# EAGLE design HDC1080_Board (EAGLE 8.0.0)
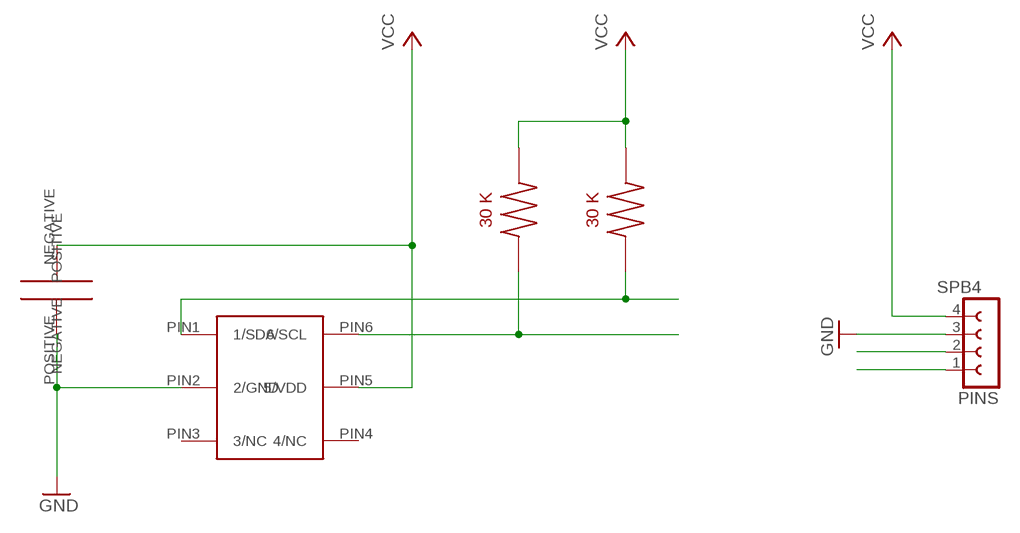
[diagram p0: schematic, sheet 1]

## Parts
PINS  SPB4  [SPB4]
U$1  HDC1080  [HDC1080]
U$2  30K_TH_RESISTOR_1135-1507  [1135-1507]
U$3  30K_TH_RESISTOR_1135-1507  [1135-1507]
U$4  CERAM_CAP_0.1UF  [CAP_CERAMIC_0.1UF]

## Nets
ONE: PINS.3 U$1.PIN2(2/GND) U$4.POSITIVE ; supply symbol labelled GND
SCL: PINS.1 U$1.PIN6(6/SCL) U$3.1
SDA: PINS.2 U$1.PIN1(1/SDA) U$2.1
VCC: PINS.4 U$1.PIN5(5/VDD) U$2.2 U$3.2 U$4.NEGATIVE
Unconnected: U$1.PIN3(3/NC) U$1.PIN4(4/NC)

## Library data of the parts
PINS = con-hirschmann:SPB4: CONNECTOR 4 pins; OC_FARNELL: unknown; OC_NEWARK: unknown
U$1 = HDC1080:HDC1080
U$2 U$3 = QBiT_Em'sComponents:30K_TH_RESISTOR_1135-1507
U$4 = Cap_Ceram_0.1uf:CERAM_CAP_0.1UF

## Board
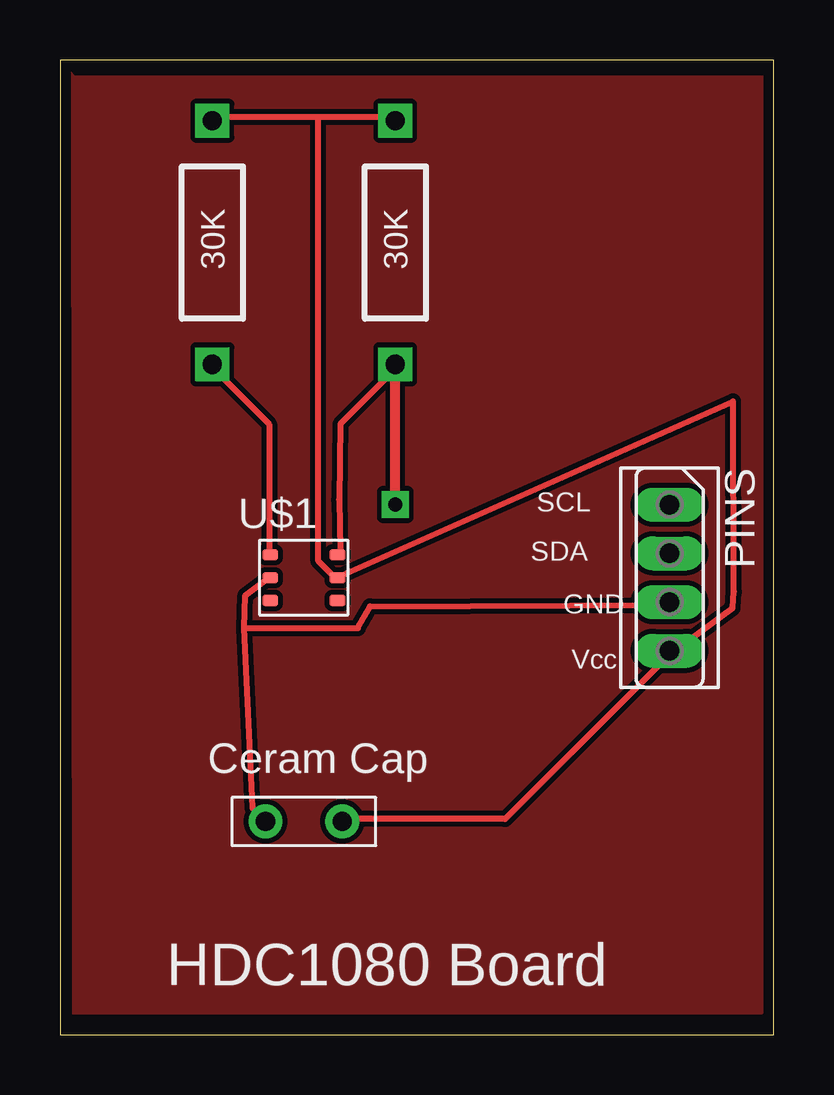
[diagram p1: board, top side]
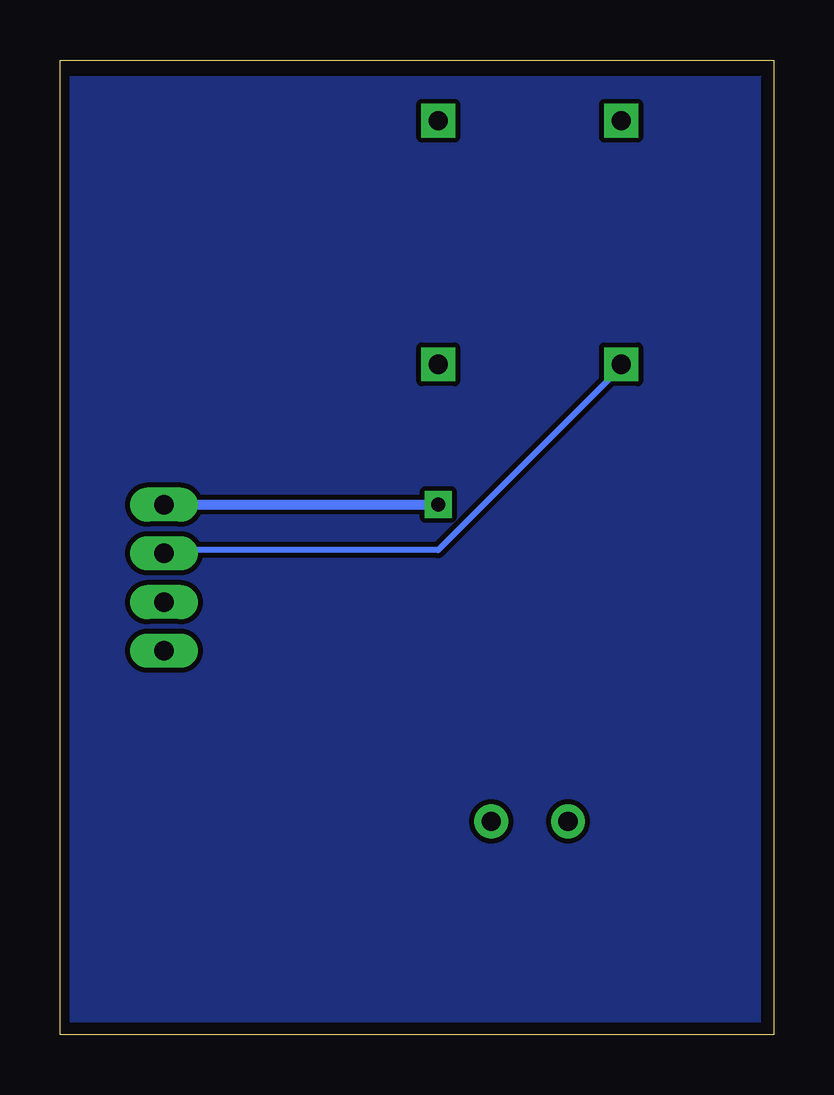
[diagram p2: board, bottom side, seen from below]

Size 29.73 x 40.63 mm. Coordinates in mm from the lower left corner, seen from the top.
Outline: 0,0 29.73,0 29.73,40.63 0,40.63 0,0
Copper layers (1*16): Top 0.035mm / dielectric 1.5mm / Bottom 0.035mm
Design rules "SparkFun": minimum track width 8mil, minimum drill 20mil, track to track 8mil, track to pad 8mil, pad to pad 8mil, via to via 8mil, smd to smd 8mil, copper to edge 10mil, drill to drill 8mil, minimum pad ring 12mil, minimum via ring 10mil, stop-mask expansion 4mil, vias tented up to drill 25mil, thermal gap 10mil

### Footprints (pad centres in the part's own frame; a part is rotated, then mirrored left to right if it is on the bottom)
SPB4 = drill 0.813 long: 1 -3.048,0; 2 -1.016,0; 3 1.016,0; 4 3.048,0
HDC1080 = smd 0.67 x 0.47: PIN1 -1.4,0.95; PIN2 -1.4,0; PIN3 -1.4,-0.95; PIN4 1.4,-0.95; PIN5 1.4,0; PIN6 1.4,0.95
1135-1507 = drill 0.8 square: 1 -5.08,0; 2 5.08,0
CAP_CERAMIC_0.1UF = drill 0.8 pad 1.25: NEGATIVE 1.6,0; POSITIVE -1.6,0

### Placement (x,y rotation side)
PINS  25.4,19.05 270 top
U$1  10.16,19.05 0 top
U$2  6.35,33.02 90 top
U$3  13.97,33.02 90 top
U$4  10.16,8.89 0 top

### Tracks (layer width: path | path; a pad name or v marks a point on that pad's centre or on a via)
GND
  pour Top (isolate 0.012): 0.46,40.11 0.51,0.86 29.26,0.86 29.26,0.91 29.31,0.91 29.31,39.96 0.61,39.96
  pour Bottom (isolate 0.012): 0.56,39.91 0.56,0.51 29.31,0.51 29.31,39.96 0.51,39.96
ONE
  Top 0.254: 7.68,16.95 8.03,9.45 8.48,8.99 U$4.POSITIVE | 7.68,16.95 7.73,18.31 8.71,19.05 U$1.PIN2 | 7.68,16.95 12.41,16.95 12.92,17.86 25.4,17.91 PINS.3
SCL  (via drill 0.6)
  Top 0.254: U$1.PIN6 11.68,20.19 11.63,22.3 11.68,25.45 13.97,27.74 U$3.1 | 25.4,22.25 PINS.1
  Top 0.406: v13.97,22.1 U$3.1
  Bottom 0.406: PINS.1 v13.97,22.1
SDA
  Top 0.254: U$1.PIN1 8.71,20.19 8.71,25.45 6.43,27.74 U$2.1
  Bottom 0.254: PINS.2 25.4,20.19 13.97,20.19 6.43,27.74 U$2.1
VCC
  Top 0.254: 10.77,38.25 13.97,38.25 U$3.2 | 10.77,38.25 6.43,38.25 U$2.2 | 25.4,15.85 28.03,17.78 28.08,18.46 28.04,26.4 U$1.PIN5 11.45,19.05 10.77,19.74 10.77,38.25 | 25.4,15.85 18.54,8.99 11.91,8.99 U$4.NEGATIVE | 25.4,15.85 PINS.4

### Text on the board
tPlace: SCL | SDA | GND | Vcc | HDC1080 Board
